{attribute 'pack_mode' := '8'} 
TYPE stAcquisitionData :
STRUCT
	(* DC Time Stamp infomation *)	
	nDcTimeStamp		: T_DCTIME;		(* Data Acquisition DC TimeStamp  *)
	(* From IO Terminal *)
	AIN0	: DINT;
	AIN1	: DINT;
	AIN2	: DINT;
	AIN3	: DINT;
	ADC_nSample			: UINT;
	ECAT_IRQ_Counter	: UINT;
	ECAT_SYNC0_Counter	: UINT;
	ECAT_SYNC1_Counter	: UINT;
END_STRUCT
END_TYPE
